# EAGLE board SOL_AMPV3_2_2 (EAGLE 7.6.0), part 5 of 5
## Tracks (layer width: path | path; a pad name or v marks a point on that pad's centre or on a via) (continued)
V5  (via drill 0.4, 0.6) (continued)
  Top 0.254: v41.97,208.47 D0:U1.3 | v88.96,206.19 88.96,204.48 D1:U1.3 | v41.97,197.04 D2:U1.3 | v88.96,194.25 88.96,192.54 D3:U1.3 | v41.97,181.8 D4:U1.3 | v88.96,179.26 D5:U1.3 | v41.97,169.1 D6:U1.3 | v88.96,167.83 D7:U1.3 | v41.97,156.4 D8:U1.3 | v88.96,155.13 D9:U1.3 | v44.51,143.06 44.51,141.36 D10:U1.3 | v88.96,142.43 D11:U1.3 | v41.97,131 D13:U1.3 | v88.96,132.27 D12:U1.3 | v41.97,118.3 D15:U1.3 | v88.96,117.03 D14:U1.3 | v41.97,101.79 D16:U1.3 | v78.17,98.87 78.17,97.17 D17:U1.3 | v41.97,90.61 41.97,88.91 D18:U1.3 | v78.17,87.44 78.17,85.74 D19:U1.3 | v43.24,75.12 43.24,73.42 D20:U1.3 | v85.15,72.58 D21:U1.3 | v41.97,63.69 D22:U1.3 | v88.96,61.15 D23:U1.3 | v41.97,48.45 D24:U1.3 | v88.96,46.42 88.96,44.72 D25:U1.3 | v41.97,37.02 D26:U1.3 | v88.96,34.99 88.96,33.29 D27:U1.3 | v42.61,23.69 42.61,21.98 D28:U1.3 | v88.96,20.77 88.96,19.06 D29:U1.3 | v42.61,12.26 42.61,10.55 D30:U1.3 | v88.96,9.08 D31:U1.3 | LED1.A v105.66,111.76
  Top 0.305: C24.1 117.93,191.77 U19.5 | R30.2 T5V.TP | U17.5 C25.1
  Top 0.406: v131.06,74.93 C25.1 | C24.1 115.82,191.75 v115.82,189.87
  Top 0.813: U21.3 T5V.TP | v101.35,111.12 C18.+ 101.35,109.83 D41.C
  Route2 0.254: v105.66,111.76 105.68,111.69
  Route2 0.305: v132.33,123.95 128.27,123.95 127.13,122.81 125.09,122.81 v122.68,119.38 | v125.73,189.99 123.19,192.53 118.49,192.53 v115.82,189.87 | v134.87,29.46 102.87,29.46 101.85,28.45 89.98,28.45 v88.96,29.46
  Route2 0.406: v88.89,111.24 89.18,111.22 91.7,111.22 | v77.73,111.37 v77.72,111.37 77.09,111.37 | v117.73,74.93 v131.06,74.93 | v115.82,189.87 96.77,189.87 96.14,189.23 v88.96,189.23
  Route2 0.813: T5V.TP 112.78,110.24 | v77.73,111.37 77.09,111.37
  Route2 1.016: 112.78,110.24 110.45,111.76 105.68,111.69 v101.35,111.12 v88.89,111.24 v77.73,111.37 | 77.09,111.37 v41.53,111.38
  Route3 0.305: v122.68,119.38 122.17,118.36 121.67,117.86 121.67,111.89 T5V.TP
  Route3 0.406: v41.97,131 41.97,134.18 | v41.97,156.4 v41.97,169.1 v41.97,181.8 v41.97,197.04 v41.97,208.47 | v88.96,206.19 v88.96,194.25 v88.96,189.23 v88.96,179.26 v88.96,167.83 v88.96,155.13 v88.96,142.43 v88.96,132.27 v88.96,117.03 | 88.89,112.4 v88.89,111.24 | v78.17,98.87 v78.17,87.44 78.23,87.38 78.23,82.68 | v85.15,72.58 85.09,72.39 | v88.96,61.15 v88.96,46.42 v88.96,34.99 v88.96,29.46 v88.96,20.77 v88.96,9.08 | T5V.TP 119.63,109.86 119.63,83.82 117.09,81.28 117.73,80.64 v117.73,74.93 | v41.97,48.45 v41.97,37.02 | v42.61,23.69 v42.61,12.26 | v44.51,143.06 43.62,143.06 43.43,143.26
  Route3 0.61: v41.97,118.3 v41.97,131 | v88.96,117.03 88.89,112.4 | v78.17,98.87 77.73,99.31 | 84.56,72.96 v85.15,72.58 | 87.57,62.29 v88.96,61.15 | 41.97,65.6 v41.97,63.69 v41.97,48.45 | 41.97,24.32 v42.61,23.69 | D8:U1.3 41.99,156.39 v41.97,156.4
  Route3 0.813: v41.97,118.3 v41.53,111.38 41.53,102.87 v41.97,101.79 v41.97,90.61 42.42,75.69 42.99,75.12 v43.24,75.12 42.42,66.04 41.97,65.6 | 41.97,134.18 43.43,142.24 43.43,143.26 43.43,153.24 D8:U1.3 | 77.73,99.31 v77.73,111.37 | 78.23,82.68 84.2,76.2 84.56,75.84 84.56,72.96 | 85.09,72.39 85.09,63.37 87.57,62.29 | v41.97,37.02 41.97,24.32
  BOTTOM 0.254: D0:R49.2 46.02,208.47 45.53,208.47 45.47,208.41 42.04,208.41 v41.97,208.47 | D1:R49.2 89.04,206.11 v88.96,206.19 | D3:R49.2 89.04,194.17 v88.96,194.25 | D2:R49.2 45.61,196.96 45.59,196.98 42.04,196.98 v41.97,197.04 | D4:R49.2 45.61,181.72 45.59,181.74 42.04,181.74 v41.97,181.8 | 42.04,169.16 v41.97,169.1 42.02,169.15 D6:R49.2 | v41.97,156.4 42.05,156.34 D8:R49.2 | v44.51,143.06 45.66,143.06 45.72,143 48.62,143 D10:R49.2 | v88.96,179.26 89.73,179.26 90.3,179.2 93.08,179.2 D5:R49.2 | v88.96,167.83 90.62,167.83 90.68,167.77 93.08,167.77 D7:R49.2 | v41.97,131 43.24,131 43.31,130.94 46.09,130.94 D13:R49.2 | v41.97,118.3 43.37,118.3 43.43,118.36 45.96,118.36 D15:R49.2 | v88.96,155.13 90.62,155.13 90.68,155.07 92.91,155.07 D9:R49.2 | v88.96,142.43 90.62,142.43 90.68,142.37 93.08,142.37 D11:R49.2 | v88.96,132.27 90.36,132.27 90.42,132.21 93.08,132.21 D12:R49.2 | D14:R49.2 89.04,116.95 v88.96,117.03 | D19:R49.2 78.99,87.38 v78.17,87.44 | D20:R49.2 43.32,75.04 v43.24,75.12 | D18:R49.2 42.05,90.54 v41.97,90.61 | D16:R49.2 42.05,101.71 v41.97,101.79 | D24:R49.2 42.05,48.37 v41.97,48.45 | D28:R49.2 42.69,23.61 v42.61,23.69 | D29:R49.2 89.04,20.69 v88.96,20.77 | D31:R49.2 89.04,9 v88.96,9.08 | D25:R49.2 89.04,46.34 v88.96,46.42 | D27:R49.2 89.04,34.91 v88.96,34.99 | D26:R49.2 42.05,36.94 v41.97,37.02 | D30:R49.2 42.69,12.18 v42.61,12.26 | D21:R49.2 85.23,72.5 v85.15,72.58 | D22:R49.2 42.05,63.61 v41.97,63.69 | D17:R49.2 78.25,98.79 v78.17,98.87 | R42.2 132.59,124.08 v132.33,123.95 | D23:R49.2 89.04,61.07 v88.96,61.15
  BOTTOM 0.305: R55.2 126.6,189.12 v125.73,189.99 | 89.04,61.1 v88.96,61.15 | R39.2 134.76,29.61 v134.87,29.46
  BOTTOM 0.406: D0:C2.2 D0:C1.2 39.75,210.06 40.39,209.42 v41.97,208.47 | D1:C2.2 D1:C1.2 86.74,207.77 87.38,207.14 v88.96,206.19 | D2:C2.2 D2:C1.2 39.75,198.63 40.39,197.99 v41.97,197.04 | D3:C2.2 D3:C1.2 86.74,195.83 87.38,195.2 v88.96,194.25 | D4:C2.2 D4:C1.2 39.75,183.39 40.39,182.75 v41.97,181.8 | D5:C2.2 D5:C1.2 86.74,180.85 87.38,180.21 v88.96,179.26 | D6:C2.2 D6:C1.2 39.75,170.69 40.39,170.05 v41.97,169.1 | D7:C2.2 D7:C1.2 86.74,169.42 87.38,168.78 v88.96,167.83 | D8:C2.2 D8:C1.2 39.75,157.99 40.39,157.35 v41.97,156.4 | D9:C2.2 D9:C1.2 86.74,156.72 87.38,156.08 v88.96,155.13 | D10:C2.2 D10:C1.2 42.29,144.65 42.93,144.02 v44.51,143.06 | D11:C2.2 D11:C1.2 86.74,144.02 87.38,143.38 v88.96,142.43 | D13:C2.2 D13:C1.2 39.75,132.59 40.39,131.95 v41.97,131 | D12:C2.2 D12:C1.2 86.74,133.86 87.38,133.22 v88.96,132.27 | D15:C2.2 D15:C1.2 39.75,119.89 40.39,119.25 v41.97,118.3 | D14:C2.2 D14:C1.2 86.74,118.62 87.38,117.98 v88.96,117.03 | D16:C2.2 D16:C1.2 39.75,103.38 40.39,102.74 v41.97,101.79 | D17:C2.2 D17:C1.2 75.95,100.46 76.58,99.82 v78.17,98.87 | D18:C2.2 D18:C1.2 39.75,92.2 40.39,91.57 v41.97,90.61 | D19:C2.2 D19:C1.2 75.95,89.03 76.58,88.39 v78.17,87.44 | D20:C2.2 D20:C1.2 41.02,76.71 41.66,76.07 v43.24,75.12 | D21:C2.2 D21:C1.2 82.93,74.17 83.57,73.53 v85.15,72.58 | D22:C2.2 D22:C1.2 39.75,65.28 40.39,64.64 v41.97,63.69 | D23:C2.2 D23:C1.2 86.74,62.74 87.38,62.1 v88.96,61.15 | D24:C2.2 D24:C1.2 39.75,50.04 40.39,49.4 v41.97,48.45 | D25:C2.2 D25:C1.2 86.74,48.01 87.38,47.37 v88.96,46.42 | D26:C2.2 D26:C1.2 39.75,38.61 40.39,37.97 v41.97,37.02 | D27:C2.2 D27:C1.2 86.74,36.58 87.38,35.94 v88.96,34.99
  BOTTOM 0.406: D28:C2.2 D28:C1.2 40.39,25.27 41.02,24.64 v42.61,23.69 | D29:C2.2 D29:C1.2 86.74,22.35 87.38,21.72 v88.96,20.77 | D30:C2.2 D30:C1.2 40.39,13.84 41.02,13.21 v42.61,12.26 | D31:C2.2 D31:C1.2 86.74,10.67 87.38,10.03 v88.96,9.08
V5D  (via drill 0.5, 0.6)
  Top 0.254: U5.7 119.38,204.98 C22.1 118.36,206.38 R51.2 v114.55,205.74 | R33.1 R49.2 | U13.7 122.17,84.84 121.54,84.84 119.89,84.84 R13.2 | U3.3 115.44,10.41 117.65,10.98 | 117.65,10.98 v118.87,12.06 | 117.65,10.98 117.98,11.31 C5.1 118.24,10.18 C8.1 121.3,10.03 121.54,9.53 122.19,8.88 R16.2
  Top 0.305: R4.2 v15.49,192.41 | U22.3 132.19,96.39 R2.2 | C6.1 U4.3 116.15,80.34 116.46,80.64 | 121.52,86.36 C23.1 121.54,84.84 | R28.2 v15.49,83.19 | R24.2 61.85,143.51 v61.47,145.16 | v16.76,32.38 14.87,32.38 R40.2 | R43.2 59.29,28.59 v59.31,28.57 | R21.2 17.02,143.64 v16.76,143.38 | v114.55,196.47 115.44,196.47 116.2,197.23 R33.1
  Top 0.406: U4.3 115.19,79.38 R47.2 | 121.52,86.36 v117.73,86.36 116.46,86.36 | 116.46,80.64 116.46,86.36 | R35.2 58.02,78.75 v58.04,78.74 | v61.21,191.77 59.93,191.77 R10.2 | R48.2 112.78,85.09 114.05,86.36 116.46,86.36
  Top 0.813: U22.3 T5D.TP | v117.73,93.98 C16.+ 116.05,91.44 D42.C
  Route2 0.305: v104.27,184.15 v114.43,184.15
  Route2 0.406: v56.77,107.95 56.77,109.22 | v61.85,107.95 61.85,109.22 | v117.73,86.36 107.44,86.36 104.39,89.41 v104.39,89.92
  Route2 0.813: T5D.TP 117.73,96.52 | 117.73,96.52 v101.98,96.96 102.28,97.16 98.68,97.16 v96.77,98.42 | v117.73,93.98 117.73,96.52 | v96.77,109.22 61.85,109.22 56.77,109.22 v16.76,109.22
  Route3 0.254: v114.55,196.47 v114.55,205.74
  Route3 0.305: v15.49,192.41 16.13,192.41 16.76,191.77 v16.76,143.38 v16.76,109.22 16.76,83.19 | 16.76,83.19 v16.76,32.38 | v15.49,83.19 16.76,83.19 | v59.31,28.57 59.31,44.32 60.2,45.21 T3.5 59.94,45.97 58.93,46.99 58.93,48.77 59.18,49.78 59.31,78.11 v58.04,78.74 | T1.5 61.85,166.88 60.58,166.88 | 104.39,179.83 v104.27,184.15 | v114.43,184.15 v114.55,196.47 | 101.85,97.08 v101.98,96.96
  Route3 0.406: v117.73,93.98 v117.73,86.36 114.55,83.19 114.55,75.18 112.65,73.28 112.65,25.4 116.08,25.4 121.67,19.81 121.67,14.86 v118.87,12.06 | v61.85,107.95 v61.47,145.16 61.47,145.8 60.58,146.69 60.58,166.88 60.58,185.42 61.85,186.69 61.85,191.13 v61.21,191.77 | v58.04,78.74 56.77,80.01 v56.77,107.95 | v104.39,89.92 104.39,94.61 102.48,96.53 v101.98,96.96 | 104.39,179.83 103.38,112.39 102.87,111.89 102.87,108.71 101.85,107.7 101.85,97.08
  Route3 0.813: v96.77,98.42 v96.77,109.22
V5E1
  Top 0.406: X4.A32 143.76,90.55 143.76,90.81 143.13,91.44 139.95,91.44 139.06,90.55 X4.C32 V5E1.TP
V5E2
  Top 0.406: V5E2.TP X3.C32 139.06,207.9 139.95,207.01 143.13,207.01 143.76,207.65 143.76,207.9 X3.A32
VBIAS  (via drill 0.4, 0.6)
  Top 0.254: D0:R36.2 25.78,209.42 25.15,210.06 v25.15,210.69 | D1:R36.2 72.77,207.14 72.14,207.77 v72.14,208.41 | D2:R36.2 25.78,197.99 25.15,198.63 v25.15,199.26 | D3:R36.2 72.77,195.2 72.14,195.83 v72.14,196.47 | D4:R36.2 25.78,182.75 25.15,183.39 v25.15,184.02 | D5:R36.2 72.77,180.21 72.14,180.85 v72.14,181.48 | D6:R36.2 25.78,170.05 25.15,170.69 v25.15,171.32 | D7:R36.2 72.77,168.78 72.14,169.42 v72.14,170.05 | D8:R36.2 25.78,157.35 25.15,157.99 v25.15,158.62 | D9:R36.2 72.77,156.08 72.14,156.72 v72.14,157.35 | D10:R36.2 28.32,144.02 27.69,144.65 v27.69,145.29 | D11:R36.2 72.77,143.38 72.14,144.02 v72.14,144.65 | D13:R36.2 25.78,131.95 25.15,132.59 v25.15,133.22 | D12:R36.2 72.77,133.22 72.14,133.86 v72.14,134.49 | D15:R36.2 25.78,119.25 25.15,119.89 v25.15,120.52 | D14:R36.2 72.77,117.98 72.14,118.62 v72.14,119.25 | D16:R36.2 25.78,102.74 25.15,103.38 v25.15,104.01 | D17:R36.2 61.98,99.82 61.34,100.46 v61.34,101.09 | D18:R36.2 25.78,91.57 25.15,92.2 v25.15,92.84 | D19:R36.2 61.98,88.39 61.34,89.03 v61.34,89.66 | D20:R36.2 27.05,76.07 26.42,76.71 v26.42,77.34 | D21:R36.2 68.96,73.53 68.33,74.17 v68.33,74.8 | D22:R36.2 25.78,64.64 25.15,65.28 v25.15,65.91 | D23:R36.2 72.77,62.1 72.14,62.74 v72.14,63.37 | D24:R36.2 25.78,49.4 25.15,50.04 v25.15,50.67 | D25:R36.2 72.77,47.37 72.14,48.01 v72.14,48.64 | D26:R36.2 25.78,37.97 25.15,38.61 v25.15,39.24 | D27:R36.2 72.77,35.94 72.14,36.58 v72.14,37.21 | D28:R36.2 26.42,24.64 25.78,25.27 v25.78,25.91 | D29:R36.2 72.77,21.72 72.14,22.35 v72.14,22.99 | D30:R36.2 26.42,13.21 25.78,13.84 v25.78,14.48 | D31:R36.2 72.77,10.03 72.14,10.67 v72.14,11.3
  Top 0.254: U3.8 112.51,11.56 | 110.43,12.7 R9.1 | 107.88,13.02 VB.TP
  Top 0.305: 112.51,11.56 111.38,12.7 110.43,12.7 | R9.1 107.88,13.02
  Route2 0.305: VB.TP 104.14,13.84 101.85,13.97 v72.01,13.97 68.83,13.97 65.66,17.14 26.29,17.14 25.65,16.51 25.65,14.61 v25.78,14.48 | v63.75,119.38 69.47,119.38
  Route2 0.406: 69.47,119.38 72.01,119.38 v72.14,119.25
  Route3 0.305: v25.15,199.26 23.75,199.39 | 23.75,199.39 23.75,209.8 v25.15,210.69 | v25.78,14.48 26.92,15.24 26.82,25.91 | 26.82,25.91 26.68,39.25 | 26.68,39.25 26.56,50.68 | 26.56,50.68 27.13,66.03 | 27.13,66.03 27.13,70.06 27.69,70.61 27.56,77.47 | 27.56,77.47 26.29,93.22 | 26.29,93.22 26.29,104.14 | 26.29,104.14 26.29,120.65 | 26.29,120.65 26.29,133.35 | 26.29,133.35 26.29,145.41 | 26.29,145.41 23.75,151.76 23.75,158.75 | 23.75,158.75 23.75,171.45 | 23.75,171.45 23.88,183.13 25.15,184.15 | 25.15,184.15 25.15,184.91 23.75,186.06 23.75,199.39 | v27.69,145.29 26.42,145.29 26.29,145.41 | v25.15,158.62 23.88,158.62 23.75,158.75 | v25.15,171.32 23.88,171.32 23.75,171.45 | v25.15,133.22 25.78,133.22 26.29,133.35 | v25.15,120.52 26.42,120.52 26.29,120.65 | 25.15,184.15 v25.15,184.02 | 26.29,104.14 25.65,104.14 v25.15,104.01 | v25.15,92.84 26.29,93.22 | 27.56,77.47 v26.42,77.34 | v25.78,25.91 26.81,25.91 26.82,25.91 | v25.15,39.24 26.67,39.24 26.68,39.25 | v25.15,50.67 26.56,50.67 26.56,50.68 | v25.15,65.91 27.01,65.91 27.13,66.03 | v72.14,11.3 72.01,13.08 v72.01,13.97 73.28,15.24 73.28,21.84 v72.14,22.99 72.14,28.07 74.55,30.48 74.55,34.8 v72.14,37.21 72.14,38.86 73.28,40.01 73.28,47.5 v72.14,48.64 72.14,54.1 73.91,55.88 73.91,61.59 v72.14,63.37 72.14,70.48 68.33,74.3 v68.33,74.8 68.33,82.68 v61.34,89.66 61.34,90.3 62.48,91.44 62.48,99.95 v61.34,101.09 61.34,103.63 63.12,105.41 63.12,118.75 v63.75,119.38 | 73.28,120.65 73.28,133.35 v72.14,134.49 72.14,135.13 72.01,135.25 72.01,135.89 73.91,137.79 73.91,142.88 v72.14,144.65 72.14,147.19 72.64,147.96 74.55,149.86 74.55,154.94 v72.14,157.35 72.14,159.51 73.28,160.66 73.28,168.58 73.2,168.91 72.9,169.29 v72.14,170.05 72.14,173.99 73.91,175.9 73.91,179.2 72.14,180.97 v72.14,181.48 72.14,187.96 73.91,189.87 73.91,194.69 v72.14,196.47 72.14,200.79 73.28,201.93 73.28,207.26 v72.14,208.41
  Route3 0.406: 73.28,120.65 73.28,120.4 v72.14,119.25
VCOMA  (via drill 0.4, 0.6)
  Top 0.305: U19.4 118.59,193.06 118.87,192.79 118.87,192.28 119.38,191.77 120.02,191.77 U19.1 119.76,191.01 119.13,190.5 v118.24,189.48
  Route2 0.305: v118.24,189.48 117.09,187.96 82.17,187.96 v81.53,188.59 | v81.66,164.66 81.66,163.32 80.9,162.56 v34.54,161.93
  Route3 0.305: v81.66,113.86 v81.66,129.09 v81.66,139.26 v81.66,151.96 v81.66,164.66 v81.66,176.09 81.66,188.47 v81.53,188.59 81.53,190.94 v81.66,191.07 v81.66,203.01 | v34.67,205.3 v34.67,193.87 v34.67,178.62 v34.67,165.93 34.54,165.8 v34.54,161.93 v34.67,153.23 37.08,151.13 v37.21,139.89 v34.67,127.83 v34.67,115.13
  BOTTOM 0.254: D0:R1.1 35.94,206.56 v34.67,205.3 | D2:R1.1 35.94,195.14 v34.67,193.87 | D4:R1.1 35.94,179.9 v34.67,178.62 | D6:R1.1 35.94,167.2 v34.67,165.93 | D8:R1.1 35.94,154.5 v34.67,153.23 | D10:R1.1 38.48,141.16 v37.21,139.89 | D13:R1.1 35.94,129.09 v34.67,127.83 | D15:R1.1 35.94,116.39 v34.67,115.13 | D14:R1.1 82.93,115.13 v81.66,113.86 | D12:R1.1 82.93,130.37 v81.66,129.09 | D11:R1.1 82.93,140.53 v81.66,139.26 | D9:R1.1 82.93,153.23 v81.66,151.96 | D1:R1.1 82.93,204.28 v81.66,203.01 | D7:R1.1 82.93,165.93 v81.66,164.66 | D3:R1.1 82.93,192.34 v81.66,191.07 | D5:R1.1 82.93,177.36 v81.66,176.09
VCOMB  (via drill 0.4, 0.6)
  Top 0.305: U17.4 128.27,71.12 128.02,71.12 127.89,71.25 127.89,71.5 127.61,71.78 U17.1 126.85,72.8 v126.62,73.03
  Route2 0.305: v126.62,73.03 101.22,73.03 95.5,78.74 v77.72,78.74 | v34.54,55.88 69.47,55.88 70.1,55.24 v81.66,55.24
  Route3 0.305: 81.53,44.45 81.53,45.72 82.17,54.74 v81.66,55.24 v81.66,57.98 81.53,58.1 81.53,62.87 77.85,66.55 v77.85,69.41 77.72,69.53 v77.72,78.74 71.37,82.55 v70.87,84.26 v70.87,95.69 | v81.66,17.59 v81.66,5.91 | v35.31,9.08 v35.31,20.51 34.67,21.14 v34.67,33.85 v34.67,45.28 34.67,55.37 v34.54,55.88 34.67,56.39 v34.67,60.52 v35.94,71.94 v34.67,87.44 v34.67,98.61
  Route3 0.406: 81.53,44.45 v81.66,43.24 v81.66,31.81 v81.66,17.59
  BOTTOM 0.254: D30:R1.1 36.58,10.35 v35.31,9.08 | D17:R1.1 72.14,96.97 v70.87,95.69 | D19:R1.1 72.14,85.53 v70.87,84.26 | D21:R1.1 79.12,70.67 v77.85,69.41 | D23:R1.1 82.93,59.24 v81.66,57.98 | D25:R1.1 82.93,44.51 v81.66,43.24 | D27:R1.1 82.93,33.08 v81.66,31.81 | D29:R1.1 82.93,18.86 v81.66,17.59 | D26:R1.1 35.94,35.12 v34.67,33.85 | D28:R1.1 36.58,21.78 v35.31,20.51 | D24:R1.1 35.94,46.55 v34.67,45.28 | D22:R1.1 35.94,61.78 v34.67,60.52 | D20:R1.1 37.21,73.22 v35.94,71.94 | D16:R1.1 35.94,99.89 v34.67,98.61 | D18:R1.1 35.94,88.71 v34.67,87.44 | D31:R1.1 82.93,7.18 v81.66,5.91
VEE  (via drill 0.4, 0.6)
  Top 0.254: v42.93,209.42 42.29,209.42 41.97,209.74 41.97,210.81 D0:U1.6 | v89.92,207.14 89.28,207.14 88.96,207.45 D1:U1.6 | v42.93,197.99 42.29,197.99 41.97,198.31 41.97,199.38 D2:U1.6 | v89.92,195.2 89.28,195.2 88.96,195.52 88.96,196.58 D3:U1.6 | v42.93,182.75 42.29,182.75 41.97,183.07 41.97,184.14 D4:U1.6 | v89.92,180.21 89.28,180.21 88.96,180.53 88.96,181.6 D5:U1.6 | v42.93,170.05 42.29,170.05 41.97,170.37 41.97,171.44 D6:U1.6 | v89.92,168.78 89.28,168.78 88.96,169.1 88.96,170.17 D7:U1.6 | v42.93,157.35 42.29,157.35 41.97,157.67 41.97,158.74 D8:U1.6 | v89.92,156.08 89.28,156.08 88.96,156.4 88.96,157.47 D9:U1.6 | v45.47,144.02 44.83,144.02 44.51,144.34 44.51,145.4 D10:U1.6 | v89.92,143.38 89.28,143.38 88.96,143.7 88.96,144.77 D11:U1.6 | v42.93,131.95 42.29,131.95 41.97,132.27 41.97,133.34 D13:U1.6 | v89.92,133.22 89.28,133.22 88.96,133.54 88.96,134.61 D12:U1.6 | v42.93,119.25 42.29,119.25 41.97,119.57 41.97,120.64 D15:U1.6 | v89.92,117.98 89.28,117.98 88.96,118.3 88.96,119.37 D14:U1.6 | v42.93,102.74 42.29,102.74 41.97,103.06 41.97,104.13 D16:U1.6 | v79.12,99.82 78.49,99.82 78.17,100.14 78.17,101.21 D17:U1.6 | v42.93,91.57 42.29,91.57 41.97,91.89 D18:U1.6 | v79.12,88.39 78.49,88.39 78.17,88.71 78.17,89.78 D19:U1.6 | v44.2,76.07 43.56,76.07 43.24,76.39 43.24,77.46 D20:U1.6 | v86.11,73.53 85.47,73.53 85.15,73.85 85.15,74.92 D21:U1.6 | v42.93,64.64 42.29,64.64 41.97,64.96 41.97,66.03 D22:U1.6 | v89.92,62.1 89.28,62.1 88.96,62.42 88.96,63.49 D23:U1.6 | v42.93,49.4 42.29,49.4 41.97,49.72 41.97,50.79 D24:U1.6 | v89.92,47.37 89.28,47.37 88.96,47.69 88.96,48.76 D25:U1.6
  Top 0.254: v42.93,37.97 42.29,37.97 41.97,38.29 41.97,39.36 D26:U1.6 | v89.92,35.94 89.28,35.94 88.96,36.26 88.96,37.33 D27:U1.6 | v43.56,24.64 42.93,24.64 42.61,24.96 42.61,26.02 D28:U1.6 | v89.92,21.72 89.28,21.72 88.96,22.04 D29:U1.6 | v43.56,13.21 42.93,13.21 42.61,13.53 42.61,14.59 D30:U1.6 | v89.92,10.03 89.28,10.03 88.96,10.35 88.96,11.42 D31:U1.6 | 123.32,121.67 123.7,121.67 U14.12 | U14.11 123.39,122.22 123.19,122.43 | U14.10 123.27,122.86 123.19,122.94
  Top 0.305: 121.85,122.86 R53.1 | U14.9 123.27,123.39 123.19,123.32
  Top 0.61: TVN3.TP 114.96,123.19 C17.- 117.12,123.42 117.84,122.7 C15.2 118.12,122.68 119.89,122.68 120.38,123.17 R53.1 121.78,122.94 123.19,122.94 | 123.19,123.32 123.19,122.94 | 123.19,122.94 123.19,122.43 123.19,121.79 123.32,121.67
  Top 0.813: D43.A v109.47,125.09
  Route2 0.813: v90.42,107.44 79.88,107.44 v79.12,99.82
  Route2 1.016: TVN3.TP 110.74,125.09 v109.47,125.09 v89.79,125.09 44.07,125.09 v43.43,126.36
  Route3 0.305: 44.07,13.97 v43.56,13.21 | v42.93,49.4 44.07,49.4 | v42.93,102.74 44.07,102.74 | v42.93,91.57 44.07,91.57 | v44.2,76.07 45.34,76.07 | v42.93,64.64 44.07,64.64 | v42.93,37.97 44.07,37.97 | v43.56,24.64 44.7,24.64 | v42.93,119.25 43.94,119.25 44.07,119.38
  Route3 0.406: 45.47,141.73 v45.47,144.02 | v42.93,157.35 v42.93,170.05 v42.93,182.75 v42.93,197.99 v42.93,209.42 | v89.92,10.03 v89.92,21.72 89.92,27.3 90.68,28.07 90.68,29.97 89.92,30.73 v89.92,35.94 v89.92,47.37 v89.92,62.1 | v89.92,207.14 v89.92,195.2 90.17,195.2 90.42,194.94 90.42,180.72 v89.92,180.21 v89.92,168.78 v89.92,156.08 v89.92,143.38 v89.92,133.22 89.92,125.22 v89.79,125.09 89.92,124.97 v89.92,117.98 90.42,117.73 | v79.12,99.82 v79.12,88.39 79.63,86.23 | 86.11,76.71 v86.11,73.53 86.61,73.26 | v42.93,131.95 44.83,131.95 44.96,132.08
  Route3 0.61: 44.07,37.97 44.07,26.04 44.7,25.4 44.7,24.64 44.7,14.61 44.07,13.97 | 45.34,155.57 v42.93,157.35 | 90.42,117.73 v90.42,107.44 | 89.66,62.87 v89.92,62.1
  Route3 0.813: 44.07,37.97 44.07,49.4 44.07,64.64 45.34,76.07 44.07,91.57 44.07,102.74 44.07,119.38 44.07,120.65 43.43,123.19 v43.43,126.36 44.96,130.43 44.96,132.08 44.96,141.22 45.47,141.73 | v45.47,144.02 45.34,155.57 | 79.63,86.23 86.11,76.71 | 86.61,73.26 87.11,66.17 89.15,63.63 89.66,62.87
  BOTTOM 0.254: D0:C4.2 D0:C3.2 41.66,210.69 v42.93,209.42 43.31,209.42 43.69,209.04 44.43,209.04 D0:R39.2 | D1:C4.2 D1:C3.2 88.65,208.41 v89.92,207.14 90.28,206.77 D1:R39.2 | D2:C4.2 D2:C3.2 41.66,199.26 v42.93,197.99 43.29,197.63 D2:R39.2 | D3:C4.2 D3:C3.2 88.65,196.47 v89.92,195.2 90.28,194.83 D3:R39.2 | D4:C4.2 D4:C3.2 41.66,184.02 v42.93,182.75 43.29,182.39 D4:R39.2 | D5:C4.2 D5:C3.2 88.65,181.48 v89.92,180.21 D5:R39.2 | D6:C4.2 D6:C3.2 41.66,171.32 v42.93,170.05 43.26,169.98 D6:R39.2 | D7:C4.2 D7:C3.2 88.65,170.05 v89.92,168.78 D7:R39.2 | D8:C4.2 D8:C3.2 41.66,158.62 v42.93,157.35 43.29,156.99 D8:R39.2 | D9:C4.2 D9:C3.2 88.65,157.35 v89.92,156.08 90.28,155.72 D9:R39.2 | D10:C4.2 D10:C3.2 44.2,145.29 v45.47,144.02 45.83,143.65 D10:R39.2 | D11:C4.2 D11:C3.2 88.65,144.65 v89.92,143.38 90.28,143.02 D11:R39.2 | D13:C4.2 D13:C3.2 41.66,133.22 v42.93,131.95 43.29,131.59 D13:R39.2 | D12:C4.2 D12:C3.2 88.65,134.49 v89.92,133.22 90.28,132.86 D12:R39.2 | D15:C4.2 D15:C3.2 41.66,120.52 v42.93,119.25 43.16,119.01 D15:R39.2 | D14:C4.2 D14:C3.2 88.65,119.25 v89.92,117.98 90.28,117.62 D14:R39.2 | D16:C4.2 D16:C3.2 41.66,104.01 v42.93,102.74 43.29,102.38 D16:R39.2 | D17:C4.2 D17:C3.2 77.85,101.09 v79.12,99.82 | D18:C4.2 D18:C3.2 41.66,92.84 v42.93,91.57 43.29,91.2 D18:R39.2 | D19:C4.2 D19:C3.2 77.85,89.66 v79.12,88.39 | D20:C4.2 D20:C3.2 42.93,77.34 v44.2,76.07 44.56,75.71 D20:R39.2 | D21:C4.2 D21:C3.2 84.84,74.8 v86.11,73.53 86.47,73.17 D21:R39.2 | D22:C4.2 D22:C3.2 41.66,65.91 v42.93,64.64 43.29,64.28 D22:R39.2 | D23:C4.2 D23:C3.2 88.65,63.37 v89.92,62.1 | D24:C4.2 D24:C3.2 41.66,50.67 v42.93,49.4 43.29,49.04 D24:R39.2
  BOTTOM 0.254: D25:C4.2 D25:C3.2 88.65,48.64 v89.92,47.37 90.28,47.01 D25:R39.2 | D26:C4.2 D26:C3.2 41.66,39.24 v42.93,37.97 43.29,37.61 D26:R39.2 | D27:C4.2 D27:C3.2 88.65,37.21 v89.92,35.94 90.28,35.58 D27:R39.2 | D28:C4.2 D28:C3.2 42.29,25.91 v43.56,24.64 43.93,24.27 D28:R39.2 | D29:C4.2 D29:C3.2 88.65,22.99 v89.92,21.72 90.28,21.35 D29:R39.2 | D30:C4.2 D30:C3.2 42.29,14.48 v43.56,13.21 43.93,12.84 D30:R39.2 | D31:C4.2 D31:C3.2 88.65,11.3 v89.92,10.03 90.28,9.67 D31:R39.2
  BOTTOM 0.305: D17:R39.2 79.63,99.44 v79.12,99.82 | v79.12,88.39 D19:R39.2 | D23:R39.2 90.28,61.74 v89.92,62.1
VIN+
  Top 0.305: 131.14,102.87 131.14,103.11 | T9.1 128.27,107.95
  Top 0.61: C3.2 118.68,112.3
  Top 0.813: F2.1 T4.TP | T4.TP 128.27,107.95 127.89,107.95 125.98,109.86 125.98,111.12 124.71,112.39 119.76,112.39 119.36,111.99 119,111.99 | U21.4 119,111.99 | 118.68,112.3 119,111.99 | T4.TP C4.+ 131.14,103.11 131.09,102.14 | 131.09,102.14 131.06,101.6 128.52,99.69 U22.4 | D44.C 131.09,102.11 131.09,102.14
  BOTTOM 0.406: R45.2 130.74,108.27 T4.TP
VIN-  (via drill 0.6)
  Top 0.254: v134.87,127.51 133.86,127.51
  Top 0.406: C28.2 132.97,115.49 132.97,115.62
  Top 1.016: F3.2 132.97,113.51 132.97,115.62 TM5.TP
  BOTTOM 0.305: R27.2 134.75,127.64 v134.87,127.51
  other vias: 116.46,127.64 118.36,127.64 125.35,126.36 126.62,126.36 126.62,120.02 124.71,120.02 125.98,123.83 125.98,121.92 129.16,120.02 121.54,120.02 124.71,128.91 127.25,128.91 117.73,125.09
  pour Top (no thermals): 124.08,130.18 129.16,130.18 129.16,117.47 124.08,117.47
  pour Top: 129.16,128.27 138.05,128.27 138.05,117.47 129.16,117.47
  pour Top (no thermals): 112.65,130.18 124.08,130.18 124.08,117.47 111.38,117.47 111.38,128.91
  pour BOTTOM (no thermals): 114.55,128.91 121.16,128.91 121.16,124.08 124.08,124.08 124.08,130.18 127.89,130.18 127.89,125.09 131.7,125.09 131.7,117.47 119.63,117.47 119.63,119.38 119,119.38 116.46,121.92 114.55,121.92
VN3EN  (via drill 0.6)
  Top 0.254: U14.5 130.01,124.16 R54.2
  Top 0.305: R54.2 131.18,124.83 v132.33,125.98
  Route3 0.305: v136.91,187.45 136.91,180.85 134.87,178.82 134.87,168.66 135.89,167.64 135.89,152.4 134.37,150.88 134.37,150.37 132.84,148.84 v132.84,130.56 132.84,126.49 v132.33,125.98
  BOTTOM 0.254: R6.1 132.41,132.48 D34.C v132.84,130.56
  BOTTOM 0.305: 132.22,126.1 v132.33,125.98 | R56.1 v136.91,187.45 | v132.33,125.98 132.33,126.49 131.83,127 131.83,127.62 R27.1 | R42.1 132.95,125.36 v132.33,125.98
VTR0  (via drill 0.4, 0.5, 0.6)
  Top 0.305: U1.9 19.43,190.37 19.3,190.5 v19.3,192.41
  Route2 0.305: v19.3,205.1 25.02,205.1 v25.15,204.98
  Route3 0.305: v19.3,192.41 v19.3,205.1
  BOTTOM 0.254: D0:R50.1 26.11,205.28 v25.15,204.98
VTR1  (via drill 0.4, 0.6)
  Top 0.305: U2.9 67.44,189.1 v68.2,189.87 | v68.2,201.93 72.01,202.56 v72.14,202.69
  Route3 0.305: v68.2,189.87 v68.2,201.93
  BOTTOM 0.254: D1:R50.1 73.1,202.99 v72.14,202.69
VTR2  (via drill 0.4, 0.5)
  Top 0.305: U1.8 v25.02,189.87
  Route3 0.305: v25.02,189.87 25.02,193.42 v25.15,193.55
  BOTTOM 0.254: D2:R50.1 26.11,193.85 v25.15,193.55
VTR3  (via drill 0.4)
  Top 0.305: U2.8 68.83,188.59 69.47,189.23 72.01,189.23 72.01,190.63 v72.14,190.75
  BOTTOM 0.254: D3:R50.1 73.1,191.06 v72.14,190.75
VTR4  (via drill 0.5)
  Top 0.305: v22.48,187.96 22.35,189.36 U1.7
  Route3 0.305: v22.48,187.96 22.48,179.71 22.48,179.07 v22.48,178.44
  BOTTOM 0.305: D4:R50.1 25.7,178.61 25.65,178.56 22.61,178.56 v22.48,178.44
VTR5  (via drill 0.6)
  Top 0.305: v70.1,187.96 68.83,187.96 68.71,188.09 U2.7
  Route3 0.305: v70.1,175.26 v70.1,187.96
  BOTTOM 0.305: D5:R50.1 72.82,176.07 72.01,175.26 v70.1,175.26
VTR6  (via drill 0.5, 0.6)
  Top 0.305: U1.6 20.93,188.87 v21.21,187.96
  Route3 0.305: v21.21,165.74 v21.21,187.96
  BOTTOM 0.305: D6:R50.1 27.05,165.74 v21.21,165.74
VTR7  (via drill 0.4, 0.6)
  Top 0.305: U2.6 67.92,187.6 v68.83,186.69
  Route3 0.305: v68.83,186.69 68.83,166.37 69.47,164.47 70.99,164.47 v72.14,164.34
  BOTTOM 0.254: D7:R50.1 73.1,164.64 v72.14,164.34
VTR8  (via drill 0.4, 0.6)
  Top 0.305: U6.9 21.97,138.94 22.35,139.32 22.35,139.57 v22.48,139.7 | v22.48,153.03 25.02,153.03 v25.15,152.91
  Route3 0.305: v22.48,139.7 v22.48,153.03
  BOTTOM 0.254: D8:R50.1 26.11,153.21 v25.15,152.91
VTR9  (via drill 0.4, 0.6)
  Top 0.305: U7.9 68.33,141.48 68.58,141.73 v68.58,142.49
  Route3 0.305: v68.58,142.49 v71.76,151.64
  BOTTOM 0.254: D9:R50.1 73.1,151.94 v71.76,151.64
VTR10  (via drill 0.4, 0.6)
  Top 0.305: U6.8 v23.11,138.43
  Route2 0.305: v23.11,138.43 v27.69,139.57
  Route3 0.305: 27.56,139.45 v27.69,139.57
  BOTTOM 0.254: D10:R50.1 28.65,139.88 v27.69,139.57
VTR11  (via drill 0.4, 0.6)
  Top 0.305: U7.8 v69.47,140.97
  Route2 0.305: v69.47,140.97 70.1,140.97 v72.14,138.94
  BOTTOM 0.254: D11:R50.1 73.1,139.24 v72.14,138.94
VTR12  (via drill 0.4, 0.6)
  Top 0.305: U6.7 21.72,137.92 22.35,137.29 v22.35,136.53
  Route3 0.305: v22.35,136.53 v22.35,127.76
  BOTTOM 0.254: D13:R50.1 26.11,127.81 v22.35,127.76
VTR13  (via drill 0.4, 0.6)
  Top 0.305: U7.7 68.33,140.46 68.58,140.21 v68.58,139.19
  Route3 0.305: v68.58,139.19 v70.74,128.27
  BOTTOM 0.254: D12:R50.1 73.1,129.08 v70.74,128.27
VTR14  (via drill 0.4, 0.6)
  Top 0.305: U6.6 20.7,136.02 v20.83,135.89
  Route3 0.305: v20.83,135.89 20.83,116.59 v22.61,114.81
  BOTTOM 0.254: D15:R50.1 26.11,115.11 v22.61,114.81
VTR15  (via drill 0.4, 0.6)
  Top 0.305: U7.6 v67.06,138.18
  Route3 0.305: v67.06,138.18 67.56,117.47 v70.23,113.54
  BOTTOM 0.254: D14:R50.1 73.1,113.84 v70.23,113.54
VTR16  (via drill 0.4, 0.6)
  Top 0.305: U9.9 22.99,77.98 23.11,78.11 v23.11,80.01
  Route3 0.305: v23.11,80.01 23.11,96.52 23.75,97.16 24.64,97.16 v25.15,97.66
  BOTTOM 0.254: D16:R50.1 26.11,98.6 v25.15,97.66
VTR17  (via drill 0.4, 0.6)
  Top 0.305: U10.9 65.15,75.44 65.41,75.69 65.41,76.45 64.9,76.96 64.9,77.09 64.64,77.34 64.64,77.85 v64.39,78.11
  Route3 0.305: v64.39,78.11 64.39,79.38 60.58,83.19 60.58,83.82 59.94,84.45 59.94,93.34 v61.59,94.36
  BOTTOM 0.254: D17:R50.1 62.31,95.68 v61.59,94.36
VTR18  (via drill 0.4, 0.6)
  Top 0.305: U9.8 24.38,77.47 25.02,79.38 v25.02,80.01
  Route3 0.305: v25.02,80.01 25.02,85.72 v25.15,86.49
  BOTTOM 0.254: D18:R50.1 26.11,87.42 v25.15,86.49
VTR19  (via drill 0.4, 0.6)
  Top 0.305: U10.8 65.79,74.93 66.29,75.44 v66.29,77.47
  Route3 0.305: v66.29,77.47 66.29,80.01 64.39,81.92 64.39,82.17 v63.88,82.68
  BOTTOM 0.254: D19:R50.1 63.58,83.61 v63.88,82.68
VTR20  (via drill 0.4, 0.6)
  Top 0.305: U9.7 22.35,76.96 22.86,76.71 22.86,75.44 v22.73,75.18
  Route3 0.305: v22.73,75.18 22.73,74.04 v26.42,71.63
  BOTTOM 0.254: D20:R50.1 27.38,71.93 v26.42,71.63
VTR21  (via drill 0.6)
  Top 0.305: U10.7 64.9,74.42 65.66,73.66 v65.66,73.03
  Route3 0.305: v65.66,73.03 65.66,71.12 v68.2,69.22
  BOTTOM 0.305: v68.2,69.22 70.06,69.22 D21:R50.1
VTR22  (via drill 0.4, 0.6)
  Top 0.305: U9.6 21.34,75.44 v21.21,74.3
  Route2 0.305: v21.84,59.69 24.64,59.69 v25.15,60.2
  Route3 0.305: v21.21,74.3 v21.84,59.69
  BOTTOM 0.254: D22:R50.1 26.11,60.5 v25.15,60.2
VTR23  (via drill 0.4, 0.6)
  Top 0.305: U10.6 63.88,72.9 v64.39,72.39
  Route3 0.305: v64.39,72.39 64.39,63.5 v71.5,56.39
  BOTTOM 0.254: D23:R50.1 73.1,57.96 v71.5,56.39
VTR24  (via drill 0.4, 0.6)
  Top 0.254: U11.9 21.72,29.08 v22.48,29.84
  Route3 0.254: v22.48,29.84 22.48,42.29 v25.15,44.96
  BOTTOM 0.254: D24:R50.1 26.11,45.26 v25.15,44.96
VTR25  (via drill 0.4, 0.6)
  Top 0.305: U12.9 66.8,23.37 v68.83,26.04
  Route3 0.305: v68.83,26.04 68.83,39.62 v72.14,42.93
  BOTTOM 0.254: D25:R50.1 73.1,43.23 v72.14,42.93
VTR26  (via drill 0.4, 0.6)
  Top 0.254: U11.8 v25.02,28.57
  Route3 0.254: v25.02,28.57 25.02,33.4 v25.15,33.53
  BOTTOM 0.254: D26:R50.1 26.11,33.83 v25.15,33.53
VTR27  (via drill 0.4, 0.6)
  Top 0.305: U12.8 68.2,22.86 v70.74,25.4
  Route3 0.305: v70.74,25.4 70.74,28.7 v72.52,30.48
  BOTTOM 0.254: D27:R50.1 73.1,31.8 v72.52,30.48
VTR28  (via drill 0.4, 0.6)
  Top 0.254: U11.7 21.72,28.07 v22.48,27.3
  Route3 0.254: v22.48,27.3 22.48,21.59 24.38,19.68 25.65,19.68 v25.78,19.56
  BOTTOM 0.254: D28:R50.1 26.75,20.5 v25.78,19.56
VTR29  (via drill 0.4, 0.6)
  Top 0.305: U12.7 69.34,22.35 v69.47,22.23
  Route3 0.305: v69.47,22.23 69.47,20.19 v71.37,18.29
  BOTTOM 0.254: D29:R50.1 73.1,17.57 v71.37,18.29
VTR30  (via drill 0.4, 0.6)
  Top 0.305: U11.6 20.07,26.54 v20.57,26.04
  Route3 0.305: v20.57,26.04 20.57,12.06 23.75,8.89 25.02,8.89 v25.15,8.76
  BOTTOM 0.254: D30:R50.1 26.75,9.07 v25.15,8.76
VTR31  (via drill 0.4, 0.6)
  Top 0.305: U12.6 65.15,20.45 v65.02,20.32
  Route2 0.305: v65.02,5.08 72.01,5.08 v72.14,4.95
  Route3 0.305: v65.02,20.32 v65.02,5.08
  BOTTOM 0.254: D31:R50.1 73.1,5.89 v72.14,4.95

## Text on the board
Top: component
Route2: layer2
Route3: layer 3
BOTTOM: bottom
tNames: SOL_AMPV3 | REV: | SERIALNR: | Universiteit Antwerpen | Wim Beaumont / (C)April 2017
bNames: SOL_AMPV3 | REV: | Universiteit Antwerpen | Wim Beaumont / (C) April 2017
